| IBS file for GS864xxxxx
| Package: standard 209pin BGA
| DQ driver is programmable
| VDD=3.3V, VDDQ can be either 2.5V or 3.3V
| Date:   23 August 2006
| Rev.:
[IBIS Ver]   3.2
[File name]   gs864xxxxx.ibs
[File Rev]   1.0
[Date]   08/23/06
[Component]   GS864018T
[Manufacturer]   GSI Technology
[Package]
|  variable   typ   min   max
R_pkg   0.2   0.1   0.5
L_pkg   3nH   1nH   5nH
C_pkg   1.5pF   1pF   3pF
[Pin]   signal_name model_name  R_pin   L_pin   C_pin
 1   NC   NC
 2   NC   NC
 3   NC   NC
 4   VDDQ   POWER
 5   VSS   GND
 6   NC   NC
 7   NC   NC
 8   DQB1   IOBUF
 9   DQB2   IOBUF
 10   VSS   GND
 11   VDDQ   POWER
 12   DQB3   IOBUF
 13   DQB4   IOBUF
 14   FT#   INBUF
 15   VDD   POWER
 16   NC   NC
 17   VSS   GND
 18   DQB5   IOBUF
 19   DQB6   IOBUF
 20   VDDQ   POWER
 21   VSS   GND
 22   DQB7   IOBUF
 23   DQB8   IOBUF
 24   DQB9   IOBUF
 25   NC   NC
 26   VSS   GND
 27   VDDQ   POWER
 28   NC   NC
 29   NC   NC
 30   NC   NC
 31   LBO#   INBUF
 32   A5   INBUF
 33   A4   INBUF
 34   A3   INBUF
 35   A2   INBUF
 36   A1   INBUF
 37   A0   INBUF
 38   A20   INBUF
 39   A19   INBUF
 40   VSS   GND
 41   VDD   POWER
 42   A18   INBUF
 43   A17   INBUF
 44   A10   INBUF
 45   A11   INBUF
 46   A12   INBUF
 47   A13   INBUF
 48   A14   INBUF
 49   A15   INBUF
 50   A16   INBUF
 51   NC   NC
 52   NC   NC
 53   NC   NC
 54   VDDQ   POWER
 55   VSS   GND
 56   NC   NC
 57   NC   NC
 58   DQA1   IOBUF
 59   DQA2   IOBUF
 60   VSS   GND
 61   VDDQ   POWER
 62   DQA3   IOBUF
 63   DQA4   IOBUF
 64   ZZ   INBUF
 65   VDD   POWER
 66   NC   NC
 67   VSS   GND
 68   DQA5   IOBUF
 69   DQA6   IOBUF
 70   VDDQ   POWER
 71   VSS   GND
 72   DQA7   IOBUF
 73   DQA8   IOBUF
 74   DQA9   IOBUF
 75   NC   NC
 76   VSS   GND
 77   VDDQ   POWER
 78   NC   NC
 79   NC   NC
 80   A21   INBUF
 81   A9   INBUF
 82   A8   INBUF
 83   ADV#   INBUF
 84   ADSP#   INBUF
 85   ADSC#   INBUF
 86   G#   INBUF
 87   BW#   INBUF
 88   GW#   INBUF
 89   CK   INBUF
 90   VSS   GND
 91   VDD   POWER
 92   E3#   INBUF
 93   BA#   INBUF
 94   BB#   INBUF
 95   NC   NC
 96   NC   NC
 97   E2   INBUF
 98   E1#   INBUF
 99   A7   INBUF
 100   A6   INBUF
[Component]   GS864032T
[Manufacturer]   GSI Technology
[Package]
|  variable   typ   min   max
R_pkg   0.2   0.1   0.5
L_pkg   3nH   1nH   5nH
C_pkg   1.5pF   1pF   3pF
[Pin]   signal_name model_name  R_pin   L_pin   C_pin
 1   NC   NC
 2   DQC8   IOBUF
 3   DQC7   IOBUF
 4   VDDQ   POWER
 5   VSS   GND
 6   DQC6   IOBUF
 7   DQC5   IOBUF
 8   DQC4   IOBUF
 9   DQC3   IOBUF
 10   VSS   GND
 11   VDDQ   POWER
 12   DQC2   IOBUF
 13   DQC1   IOBUF
 14   FT#   INBUF
 15   VDD   POWER
 16   NC   NC
 17   VSS   GND
 18   DQD1   IOBUF
 19   DQD2   IOBUF
 20   VDDQ   POWER
 21   VSS   GND
 22   DQD3   IOBUF
 23   DQD4   IOBUF
 24   DQD5   IOBUF
 25   DQD6   IOBUF
 26   VSS   GND
 27   VDDQ   POWER
 28   DQD7   IOBUF
 29   DQD8   IOBUF
 30   NC   NC
 31   LBO#   INBUF
 32   A5   INBUF
 33   A4   INBUF
 34   A3   INBUF
 35   A2   INBUF
 36   A1   INBUF
 37   A0   INBUF
 38   A20   INBUF
 39   A19   INBUF
 40   VSS   GND
 41   VDD   POWER
 42   A18   INBUF
 43   A17   INBUF
 44   A10   INBUF
 45   A11   INBUF
 46   A12   INBUF
 47   A13   INBUF
 48   A14   INBUF
 49   A15   INBUF
 50   A16   INBUF
 51   NC   NC
 52   DQA8   IOBUF
 53   DQA7   IOBUF
 54   VDDQ   POWER
 55   VSS   GND
 56   DQA6   IOBUF
 57   DQA5   IOBUF
 58   DQA4   IOBUF
 59   DQA3   IOBUF
 60   VSS   GND
 61   VDDQ   POWER
 62   DQA2   IOBUF
 63   DQA1   IOBUF
 64   ZZ   INBUF
 65   VDD   POWER
 66   NC   NC
 67   VSS   GND
 68   DQB1   IOBUF
 69   DQB2   IOBUF
 70   VDDQ   POWER
 71   VSS   GND
 72   DQB3   IOBUF
 73   DQB4   IOBUF
 74   DQB5   IOBUF
 75   DQB6   IOBUF
 76   VSS   GND
 77   VDDQ   POWER
 78   DQB7   IOBUF
 79   DQB8   IOBUF
 80   NC   NC
 81   A9   INBUF
 82   A8   INBUF
 83   ADV#   INBUF
 84   ADSP#   INBUF
 85   ADSC#   INBUF
 86   G#   INBUF
 87   BW#   INBUF
 88   GW#   INBUF
 89   CK   INBUF
 90   VSS   GND
 91   VDD   POWER
 92   E3#   INBUF
 93   BA#   INBUF
 94   BB#   INBUF
 95   BC#   INBUF
 96   BD#   INBUF
 97   E2   INBUF
 98   E1#   INBUF
 99   A7   INBUF
 100   A6   INBUF
[Component]   GS864036t
[Manufacturer]   GSI Technology
[Package]
|  variable   typ   min   max
R_pkg   0.2   0.1   0.5
L_pkg   3nH   1nH   5nH
C_pkg   1.5pF   1pF   3pF
[Pin]   signal_name model_name  R_pin   L_pin   C_pin
 1   DQC9   IOBUF
 2   DQC8   IOBUF
 3   DQC7   IOBUF
 4   VDDQ   POWER
 5   VSS   GND
 6   DQC6   IOBUF
 7   DQC5   IOBUF
 8   DQC4   IOBUF
 9   DQC3   IOBUF
 10   VSS   GND
 11   VDDQ   POWER
 12   DQC2   IOBUF
 13   DQC1   IOBUF
 14   FT#   INBUF
 15   VDD   POWER
 16   NC   NC
 17   VSS   GND
 18   DQD1   IOBUF
 19   DQD2   IOBUF
 20   VDDQ   POWER
 21   VSS   GND
 22   DQD3   IOBUF
 23   DQD4   IOBUF
 24   DQD5   IOBUF
 25   DQD6   IOBUF
 26   VSS   GND
 27   VDDQ   POWER
 28   DQD7   IOBUF
 29   DQD8   IOBUF
 30   DQD9   IOBUF
 31   LBO#   INBUF
 32   A5   INBUF
 33   A4   INBUF
 34   A3   INBUF
 35   A2   INBUF
 36   A1   INBUF
 37   A0   INBUF
 38   A20   INBUF
 39   A19   INBUF
 40   VSS   GND
 41   VDD   POWER
 42   A18   INBUF
 43   A17   INBUF
 44   A10   INBUF
 45   A11   INBUF
 46   A12   INBUF
 47   A13   INBUF
 48   A14   INBUF
 49   A15   INBUF
 50   A16   INBUF
 51   DQA9   IOBUF
 52   DQA8   IOBUF
 53   DQA7   IOBUF
 54   VDDQ   POWER
 55   VSS   GND
 56   DQA6   IOBUF
 57   DQA5   IOBUF
 58   DQA4   IOBUF
 59   DQA3   IOBUF
 60   VSS   GND
 61   VDDQ   POWER
 62   DQA2   IOBUF
 63   DQA1   IOBUF
 64   ZZ   INBUF
 65   VDD   POWER
 66   NC   NC
 67   VSS   GND
 68   DQB1   IOBUF
 69   DQB2   IOBUF
 70   VDDQ   POWER
 71   VSS   GND
 72   DQB3   IOBUF
 73   DQB4   IOBUF
 74   DQB5   IOBUF
 75   DQB6   IOBUF
 76   VSS   GND
 77   VDDQ   POWER
 78   DQB7   IOBUF
 79   DQB8   IOBUF
 80   DQB9   IOBUF
 81   A9   INBUF
 82   A8   INBUF
 83   ADV#   INBUF
 84   ADSP#   INBUF
 85   ADSC#   INBUF
 86   G#   INBUF
 87   BW#   INBUF
 88   GW#   INBUF
 89   CK   INBUF
 90   VSS   GND
 91   VDD   POWER
 92   E3#   INBUF
 93   BA#   INBUF
 94   BB#   INBUF
 95   BC#   INBUF
 96   BD#   INBUF
 97   E2   INBUF
 98   E1#   INBUF
 99   A7   INBUF
 100   A6   INBUF
[Component]   GS8640E18T
[Manufacturer]   GSI Technology
[Package]
|  variable   typ   min   max
R_pkg   0.2   0.1   0.5
L_pkg   3nH   1nH   5nH
C_pkg   1.5pF   1pF   3pF
[Pin]   signal_name model_name  R_pin   L_pin   C_pin
 1   NC   NC
 2   NC   NC
 3   NC   NC
 4   VDDQ   POWER
 5   VSS   GND
 6   NC   NC
 7   NC   NC
 8   DQB1   IOBUF
 9   DQB2   IOBUF
 10   VSS   GND
 11   VDDQ   POWER
 12   DQB3   IOBUF
 13   DQB4   IOBUF
 14   FT#   INBUF
 15   VDD   POWER
 16   NC   NC
 17   VSS   GND
 18   DQB5   IOBUF
 19   DQB6   IOBUF
 20   VDDQ   POWER
 21   VSS   GND
 22   DQB7   IOBUF
 23   DQB8   IOBUF
 24   DQB9   IOBUF
 25   NC   NC
 26   VSS   GND
 27   VDDQ   POWER
 28   NC   NC
 29   NC   NC
 30   NC   NC
 31   LBO#   INBUF
 32   A5   INBUF
 33   A4   INBUF
 34   A3   INBUF
 35   A2   INBUF
 36   A1   INBUF
 37   A0   INBUF
 38   A20   INBUF
 39   A19   INBUF
 40   VSS   GND
 41   VDD   POWER
 42   A18   INBUF
 43   A17   INBUF
 44   A10   INBUF
 45   A11   INBUF
 46   A12   INBUF
 47   A13   INBUF
 48   A14   INBUF
 49   A15   INBUF
 50   A16   INBUF
 51   NC   NC
 52   NC   NC
 53   NC   NC
 54   VDDQ   POWER
 55   VSS   GND
 56   NC   NC
 57   NC   NC
 58   DQA1   IOBUF
 59   DQA2   IOBUF
 60   VSS   GND
 61   VDDQ   POWER
 62   DQA3   IOBUF
 63   DQA4   IOBUF
 64   ZZ   INBUF
 65   VDD   POWER
 66   NC   NC
 67   VSS   GND
 68   DQA5   IOBUF
 69   DQA6   IOBUF
 70   VDDQ   POWER
 71   VSS   GND
 72   DQA7   IOBUF
 73   DQA8   IOBUF
 74   DQA9   IOBUF
 75   NC   NC
 76   VSS   GND
 77   VDDQ   POWER
 78   NC   NC
 79   NC   NC
 80   A21   INBUF
 81   A9   INBUF
 82   A8   INBUF
 83   ADV#   INBUF
 84   ADSP#   INBUF
 85   ADSC#   INBUF
 86   G#   INBUF
 87   BW#   INBUF
 88   GW#   INBUF
 89   CK   INBUF
 90   VSS   GND
 91   VDD   POWER
 92   E3#   INBUF
 93   BA#   INBUF
 94   BB#   INBUF
 95   NC   NC
 96   NC   NC
 97   E2   INBUF
 98   E1#   INBUF
 99   A7   INBUF
 100   A6   INBUF
[Component]   GS8640E32T
[Manufacturer]   GSI Technology
[Package]
|  variable   typ   min   max
R_pkg   0.2   0.1   0.5
L_pkg   3nH   1nH   5nH
C_pkg   1.5pF   1pF   3pF
[Pin]   signal_name model_name  R_pin   L_pin   C_pin
 1   NC   NC
 2   DQC8   IOBUF
 3   DQC7   IOBUF
 4   VDDQ   POWER
 5   VSS   GND
 6   DQC6   IOBUF
 7   DQC5   IOBUF
 8   DQC4   IOBUF
 9   DQC3   IOBUF
 10   VSS   GND
 11   VDDQ   POWER
 12   DQC2   IOBUF
 13   DQC1   IOBUF
 14   FT#   INBUF
 15   VDD   POWER
 16   NC   NC
 17   VSS   GND
 18   DQD1   IOBUF
 19   DQD2   IOBUF
 20   VDDQ   POWER
 21   VSS   GND
 22   DQD3   IOBUF
 23   DQD4   IOBUF
 24   DQD5   IOBUF
 25   DQD6   IOBUF
 26   VSS   GND
 27   VDDQ   POWER
 28   DQD7   IOBUF
 29   DQD8   IOBUF
 30   NC   NC
 31   LBO#   INBUF
 32   A5   INBUF
 33   A4   INBUF
 34   A3   INBUF
 35   A2   INBUF
 36   A1   INBUF
 37   A0   INBUF
 38   A20   INBUF
 39   A19   INBUF
 40   VSS   GND
 41   VDD   POWER
 42   A18   INBUF
 43   A17   INBUF
 44   A10   INBUF
 45   A11   INBUF
 46   A12   INBUF
 47   A13   INBUF
 48   A14   INBUF
 49   A15   INBUF
 50   A16   INBUF
 51   NC   NC
 52   DQA8   IOBUF
 53   DQA7   IOBUF
 54   VDDQ   POWER
 55   VSS   GND
 56   DQA6   IOBUF
 57   DQA5   IOBUF
 58   DQA4   IOBUF
 59   DQA3   IOBUF
 60   VSS   GND
 61   VDDQ   POWER
 62   DQA2   IOBUF
 63   DQA1   IOBUF
 64   ZZ   INBUF
 65   VDD   POWER
 66   NC   NC
 67   VSS   GND
 68   DQB1   IOBUF
 69   DQB2   IOBUF
 70   VDDQ   POWER
 71   VSS   GND
 72   DQB3   IOBUF
 73   DQB4   IOBUF
 74   DQB5   IOBUF
 75   DQB6   IOBUF
 76   VSS   GND
 77   VDDQ   POWER
 78   DQB7   IOBUF
 79   DQB8   IOBUF
 80   NC   NC
 81   A9   INBUF
 82   A8   INBUF
 83   ADV#   INBUF
 84   ADSP#   INBUF
 85   ADSC#   INBUF
 86   G#   INBUF
 87   BW#   INBUF
 88   GW#   INBUF
 89   CK   INBUF
 90   VSS   GND
 91   VDD   POWER
 92   E3#   INBUF
 93   BA#   INBUF
 94   BB#   INBUF
 95   BC#   INBUF
 96   BD#   INBUF
 97   E2   INBUF
 98   E1#   INBUF
 99   A7   INBUF
 100   A6   INBUF
[Component]   GS8640E36t
[Manufacturer]   GSI Technology
[Package]
|  variable   typ   min   max
R_pkg   0.2   0.1   0.5
L_pkg   3nH   1nH   5nH
C_pkg   1.5pF   1pF   3pF
[Pin]   signal_name model_name  R_pin   L_pin   C_pin
 1   DQC9   IOBUF
 2   DQC8   IOBUF
 3   DQC7   IOBUF
 4   VDDQ   POWER
 5   VSS   GND
 6   DQC6   IOBUF
 7   DQC5   IOBUF
 8   DQC4   IOBUF
 9   DQC3   IOBUF
 10   VSS   GND
 11   VDDQ   POWER
 12   DQC2   IOBUF
 13   DQC1   IOBUF
 14   FT#   INBUF
 15   VDD   POWER
 16   NC   NC
 17   VSS   GND
 18   DQD1   IOBUF
 19   DQD2   IOBUF
 20   VDDQ   POWER
 21   VSS   GND
 22   DQD3   IOBUF
 23   DQD4   IOBUF
 24   DQD5   IOBUF
 25   DQD6   IOBUF
 26   VSS   GND
 27   VDDQ   POWER
 28   DQD7   IOBUF
 29   DQD8   IOBUF
 30   DQD9   IOBUF
 31   LBO#   INBUF
 32   A5   INBUF
 33   A4   INBUF
 34   A3   INBUF
 35   A2   INBUF
 36   A1   INBUF
 37   A0   INBUF
 38   A20   INBUF
 39   A19   INBUF
 40   VSS   GND
 41   VDD   POWER
 42   A18   INBUF
 43   A17   INBUF
 44   A10   INBUF
 45   A11   INBUF
 46   A12   INBUF
 47   A13   INBUF
 48   A14   INBUF
 49   A15   INBUF
 50   A16   INBUF
 51   DQA9   IOBUF
 52   DQA8   IOBUF
 53   DQA7   IOBUF
 54   VDDQ   POWER
 55   VSS   GND
 56   DQA6   IOBUF
 57   DQA5   IOBUF
 58   DQA4   IOBUF
 59   DQA3   IOBUF
 60   VSS   GND
 61   VDDQ   POWER
 62   DQA2   IOBUF
 63   DQA1   IOBUF
 64   ZZ   INBUF
 65   VDD   POWER
 66   NC   NC
 67   VSS   GND
 68   DQB1   IOBUF
 69   DQB2   IOBUF
 70   VDDQ   POWER
 71   VSS   GND
 72   DQB3   IOBUF
 73   DQB4   IOBUF
 74   DQB5   IOBUF
 75   DQB6   IOBUF
 76   VSS   GND
 77   VDDQ   POWER
 78   DQB7   IOBUF
 79   DQB8   IOBUF
 80   DQB9   IOBUF
 81   A9   INBUF
 82   A8   INBUF
 83   ADV#   INBUF
 84   ADSP#   INBUF
 85   ADSC#   INBUF
 86   G#   INBUF
 87   BW#   INBUF
 88   GW#   INBUF
 89   CK   INBUF
 90   VSS   GND
 91   VDD   POWER
 92   E3#   INBUF
 93   BA#   INBUF
 94   BB#   INBUF
 95   BC#   INBUF
 96   BD#   INBUF
 97   E2   INBUF
 98   E1#   INBUF
 99   A7   INBUF
 100   A6   INBUF
[Component]   GS864218B
[Manufacturer]   GSI Technology
[Package]
|  variable   typ   min   max
R_pkg   0.2   0.1   0.5
L_pkg   3nH   1nH   5nH
C_pkg   1.5pF   1pF   3pF
[Pin]   signal_name model_name  R_pin   L_pin   C_pin
 A1   VDDQ   POWER
 A2   A6   INBUF
 A3   A7   INBUF
 A4   ADSP#   INBUF
 A5   A8   INBUF
 A6   A9   INBUF
 A7   VDDQ   POWER
 B1   NC   NC
 B2   A18   INBUF
 B3   A4   INBUF
 B4   ADSC#   INBUF
 B5   A15   INBUF
 B6   A17   INBUF
 B7   NC   NC
 C1   NC   NC
 C2   A5   INBUF
 C3   A3   INBUF
 C4   VDD   POWER
 C5   A14   INBUF
 C6   A16   INBUF
 C7   NC   NC
 D1   DQB1   Progbuf1
 D2   NC   NC
 D3   VSS   GND
 D4   ZQ   INBUF
 D5   VSS   GND
 D6   DQA9   Progbuf1
 D7   NC   NC
 E1   NC   NC
 E2   DQB2   Progbuf1
 E3   VSS   GND
 E4   E1#   INBUF
 E5   VSS   GND
 E6   NC   NC
 E7   DQA8   Progbuf1
 F1   VDDQ   POWER
 F2   NC   NC
 F3   VSS   GND
 F4   G#   INBUF
 F5   VSS   GND
 F6   DQA7   Progbuf1
 F7   VDDQ   POWER
 G1   NC   NC
 G2   DQB3   Progbuf1
 G3   BB#   INBUF
 G4   ADV#   INBUF
 G5   NC   NC
 G6   NC   NC
 G7   DQA6   Progbuf1
 H1   DQB4   Progbuf1
 H2   NC   NC
 H3   VSS   GND
 H4   GW#   INBUF
 H5   VSS   GND
 H6   DQA5   Progbuf1
 H7   NC   NC
 J1   VDDQ   POWER
 J2   VDD   POWER
 J3   NC   NC
 J4   VDD   POWER
 J5   NC   NC
 J6   VDD   POWER
 J7   VDDQ   POWER
 K1   NC   NC
 K2   DQB5   Progbuf1
 K3   VSS   GND
 K4   CK   INBUF
 K5   VSS   GND
 K6   NC   NC
 K7   DQA4   Progbuf1
 L1   DQB6   Progbuf1
 L2   NC   NC
 L3   NC   NC
 L4   SCD   INBUF
 L5   BA#   INBUF
 L6   DQA3   Progbuf1
 L7   NC   NC
 M1   VDDQ   POWER
 M2   DQB7   Progbuf1
 M3   VSS   GND
 M4   BW#   INBUF
 M5   VSS   GND
 M6   NC   NC
 M7   VDDQ   POWER
 N1   DQB8   Progbuf1
 N2   NC   NC
 N3   VSS   GND
 N4   A1   INBUF
 N5   VSS   GND
 N6   DQA2   Progbuf1
 N7   NC   NC
 P1   NC   NC
 P2   DQB9   Progbuf1
 P3   VSS   GND
 P4   A0   INBUF
 P5   VSS   GND
 P6   NC   NC
 P7   DQA1   Progbuf1
 R1   NC   NC
 R2   A2   INBUF
 R3   LBO#   INBUF
 R4   VDD   POWER
 R5   FT#   INBUF
 R6   A13   INBUF
 R7   NC   NC
 T1   A20   INBUF
 T2   A10   INBUF
 T3   A11   INBUF
 T4   A21   INBUF
 T5   A12   INBUF
 T6   A19   INBUF
 T7   ZZ   INBUF
 U1   VDDQ   POWER
 U2   TMS   INBUF
 U3   TDI   INBUF
 U4   TCK   INBUF
 U5   TDO   Progbuf2
 U6   NC   NC
 U7   VDDQ   POWER
[Component]   GS864236B
[Manufacturer]   GSI Technology
[Package]
|  variable   typ   min   max
R_pkg   0.2   0.1   0.5
L_pkg   3nH   1nH   5nH
C_pkg   1.5pF   1pF   3pF
[Pin]   signal_name model_name  R_pin   L_pin   C_pin
 A1   VDDQ   POWER
 A2   A6   INBUF
 A3   A7   INBUF
 A4   ADSP#   INBUF
 A5   A8   INBUF
 A6   A9   INBUF
 A7   VDDQ   POWER
 B1   NC   NC
 B2   A18   INBUF
 B3   A4   INBUF
 B4   ADSC#   INBUF
 B5   A15   INBUF
 B6   A17   INBUF
 B7   NC   NC
 C1   NC   NC
 C2   A5   INBUF
 C3   A3   INBUF
 C4   VDD   POWER
 C5   A14   INBUF
 C6   A16   INBUF
 C7   NC   NC
 D1   DQc4   Progbuf1
 D2   DQC9   Progbuf1
 D3   VSS   GND
 D4   ZQ   INBUF
 D5   VSS   GND
 D6   DQB9   Progbuf1
 D7   DQB4   Progbuf1
 E1   DQc3   Progbuf1
 E2   DQC8   Progbuf1
 E3   VSS   GND
 E4   E1#   INBUF
 E5   VSS   GND
 E6   DQB8   Progbuf1
 E7   DQB3   Progbuf1
 F1   VDDQ   POWER
 F2   DQC7   Progbuf1
 F3   VSS   GND
 F4   G#   INBUF
 F5   VSS   GND
 F6   DQB7   Progbuf1
 F7   VDDQ   POWER
 G1   DQc2   Progbuf1
 G2   DQC6   Progbuf1
 G3   BC#   INBUF
 G4   ADV#   INBUF
 G5   BB#   INBUF
 G6   DQB6   Progbuf1
 G7   DQB2   Progbuf1
 H1   DQc1   Progbuf1
 H2   DQC5   Progbuf1
 H3   VSS   GND
 H4   GW#   INBUF
 H5   VSS   GND
 H6   DQB5   Progbuf1
 H7   DQB1   Progbuf1
 J1   VDDQ   POWER
 J2   VDD   POWER
 J3   NC   NC
 J4   VDD   POWER
 J5   NC   NC
 J6   VDD   POWER
 J7   VDDQ   POWER
 K1   DQD1   Progbuf1
 K2   DQD5   Progbuf1
 K3   VSS   GND
 K4   CK   INBUF
 K5   VSS   GND
 K6   DQA5   Progbuf1
 K7   DQA1   Progbuf1
 L1   DQD2   Progbuf1
 L2   DQD6   Progbuf1
 L3   BD#   INBUF
 L4   SCD   INBUF
 L5   BA#   INBUF
 L6   DQA6   Progbuf1
 L7   DQA2   Progbuf1
 M1   VDDQ   POWER
 M2   DQD7   Progbuf1
 M3   VSS   GND
 M4   BW#   INBUF
 M5   VSS   GND
 M6   DQA7   Progbuf1
 M7   VDDQ   POWER
 N1   DQD3   Progbuf1
 N2   DQD8   Progbuf1
 N3   VSS   GND
 N4   A1   INBUF
 N5   VSS   GND
 N6   DQA8   Progbuf1
 N7   DQA3   Progbuf1
 P1   DQD4   Progbuf1
 P2   DQD9   Progbuf1
 P3   VSS   GND
 P4   A0   INBUF
 P5   VSS   GND
 P6   DQA9   Progbuf1
 P7   DQA4   Progbuf1
 R1   NC   NC
 R2   A2   INBUF
 R3   LBO#   INBUF
 R4   VDD   POWER
 R5   FT#   INBUF
 R6   A13   INBUF
 R7   NC   NC
 T1   NC   NC
 T2   A20   INBUF
 T3   A10   INBUF
 T4   A11   INBUF
 T5   A12   INBUF
 T6   A20   INBUF
 T7   ZZ   INBUF
 U1   VDDQ   POWER
 U2   TMS   INBUF
 U3   TDI   INBUF
 U4   TCK   INBUF
 U5   TDO   Progbuf2
 U6   NC   NC
 U7   VDDQ   POWER
[Component]   GS864272C
[Manufacturer]   GSI Technology
[Package]
|  variable   typ   min   max
R_pkg   0.2   0.1   0.5
L_pkg   3nH   1nH   5nH
C_pkg   1.5pF   1pF   3pF
[Pin]   signal_name model_name  R_pin   L_pin   C_pin
 A1   DQG5   Progbuf1
 A2   DQG1   Progbuf1
 A3   A15   INBUF
 A4   E2   INBUF
 A5   ADSP   INBUF
 A6   ADSC   INBUF
 A7   ADV   INBUF
 A8   E3   INBUF
 A9   A17   INBUF
 A10   DQB1   Progbuf1
 A11   DQB5   Progbuf1
 B1   DQG6   Progbuf1
 B2   DQG2   Progbuf1
 B3   BC   INBUF
 B4   BG   INBUF
 B5   NC   NC
 B6   BW   INBUF
 B7   A16   INBUF
 B8   BB   INBUF
 B9   BF   INBUF
 B10   DQB2   Progbuf1
 B11   DQB6   Progbuf1
 C1   DQG7   Progbuf1
 C2   DQG3   Progbuf1
 C3   BH   INBUF
 C4   BD   INBUF
 C5   NC   NC
 C6   E1   INBUF
 C7   NC   NC
 C8   BE   INBUF
 C9   BA   INBUF
 C10   DQB3   Progbuf1
 C11   DQB7   Progbuf1
 D1   DQG8   Progbuf1
 D2   DQG4   Progbuf1
 D3   VSS   GND
 D4   NC   NC
 D5   NC   NC
 D6   G   INBUF
 D7   GW   INBUF
 D8   NC   NC
 D9   VSS   GND
 D10   DQB4   Progbuf1
 D11   DQB8   Progbuf1
 E1   DQG9   Progbuf1
 E2   DQC9   Progbuf1
 E3   VDDQ   POWER
 E4   VDDQ   POWER
 E5   VDD   POWER
 E6   VDD   POWER
 E7   VDD   POWER
 E8   VDDQ   POWER
 E9   VDDQ   POWER
 E10   DQF9   Progbuf1
 E11   DQB9   Progbuf1
 F1   DQC4   Progbuf1
 F2   DQC8   Progbuf1
 F3   VSS   GND
 F4   VSS   GND
 F5   VSS   GND
 F6   ZQ   INBUF
 F7   VSS   GND
 F8   VSS   GND
 F9   VSS   GND
 F10   DQF8   Progbuf1
 F11   DQF4   Progbuf1
 G1   DQC3   Progbuf1
 G2   DQC7   Progbuf1
 G3   VDDQ   POWER
 G4   VDDQ   POWER
 G5   VDD   POWER
 G6   MCH   INBUF
 G7   VDD   POWER
 G8   VDDQ   POWER
 G9   VDDQ   POWER
 G10   DQF7   Progbuf1
 G11   DQF3   Progbuf1
 H1   DQC2   Progbuf1
 H2   DQC6   Progbuf1
 H3   VSS   GND
 H4   VSS   GND
 H5   VSS   GND
 H6   MCL   INBUF
 H7   VSS   GND
 H8   VSS   GND
 H9   VSS   GND
 H10   DQF6   Progbuf1
 H11   DQF2   Progbuf1
 J1   DQC1   Progbuf1
 J2   DQC5   Progbuf1
 J3   VDDQ   POWER
 J4   VDDQ   POWER
 J5   VDD   POWER
 J6   MCL   INBUF
 J7   VDD   POWER
 J8   VDDQ   POWER
 J9   VDDQ   POWER
 J10   DQF5   Progbuf1
 J11   DQF1   Progbuf1
 K1   NC   NC
 K2   NC   NC
 K3   CK   INBUF
 K4   NC   NC
 K5   VSS   GND
 K6   MCL   INBUF
 K7   VSS   GND
 K8   NC   NC
 K9   NC   NC
 K10   NC   NC
 K11   NC   NC
 L1   DQH1   Progbuf1
 L2   DQH5   Progbuf1
 L3   VDDQ   POWER
 L4   VDDQ   POWER
 L5   VDD   POWER
 L6   FT   INBUF
 L7   VDD   POWER
 L8   VDDQ   POWER
 L9   VDDQ   POWER
 L10   DQA5   Progbuf1
 L11   DQA1   Progbuf1
 M1   DQH2   Progbuf1
 M2   DQH6   Progbuf1
 M3   VSS   GND
 M4   VSS   GND
 M5   VSS   GND
 M6   MCL   INBUF
 M7   VSS   GND
 M8   VSS   GND
 M9   VSS   GND
 M10   DQA6   Progbuf1
 M11   DQA2   Progbuf1
 N1   DQH3   Progbuf1
 N2   DQH7   Progbuf1
 N3   VDDQ   POWER
 N4   VDDQ   POWER
 N5   VDD   POWER
 N6   SCD   INBUF
 N7   VDD   POWER
 N8   VDDQ   POWER
 N9   VDDQ   POWER
 N10   DQA7   Progbuf1
 N11   DQA3   Progbuf1
 P1   DQH4   Progbuf1
 P2   DQH8   Progbuf1
 P3   VSS   GND
 P4   VSS   GND
 P5   VSS   GND
 P6   ZZ   INBUF
 P7   VSS   GND
 P8   VSS   GND
 P9   VSS   GND
 P10   DQA8   Progbuf1
 P11   DQA4   Progbuf1
 R1   DQD9   Progbuf1
 R2   DQH9   Progbuf1
 R3   VDDQ   POWER
 R4   VDDQ   POWER
 R5   VDD   POWER
 R6   VDD   POWER
 R7   VDD   POWER
 R8   VDDQ   POWER
 R9   VDDQ   POWER
 R10   DQA9   Progbuf1
 R11   DQE9   Progbuf1
 T1   DQD8   Progbuf1
 T2   DQD4   Progbuf1
 T3   VSS   GND
 T4   NC   NC
 T5   NC   NC
 T6   LBO   INBUF
 T7   NC   NC
 T8   NC   NC
 T9   VSS   GND
 T10   DQE4   Progbuf1
 T11   DQE8   Progbuf1
 U1   DQD7   Progbuf1
 U2   DQD3   Progbuf1
 U3   A19   INBUF
 U4   A14   INBUF
 U5   A13   INBUF
 U6   A12   INBUF
 U7   A11   INBUF
 U8   A10   INBUF
 U9   A18   INBUF
 U10   DQE3   Progbuf1
 U11   DQE7   Progbuf1
 V1   DQD6   Progbuf1
 V2   DQD2   Progbuf1
 V3   A9   INBUF
 V4   A8   INBUF
 V5   A7   INBUF
 V6   A1   INBUF
 V7   A6   INBUF
 V8   A5   INBUF
 V9   A4   INBUF
 V10   DQE2   Progbuf1
 V11   DQE6   Progbuf1
 W1   DQD5   Progbuf1
 W2   DQD1   Progbuf1
 W3   TMS   INBUF
 W4   TDI   INBUF
 W5   A3   INBUF
 W6   A0   INBUF
 W7   A2   INBUF
 W8   TDO   Progbuf2
 W9   TCK   INBUF
 W10   DQE1   Progbuf1
 W11   DQE5   Progbuf1
[Component]   GS8640FZ18T
[Manufacturer]   GSI Technology
[Package]
|  variable   typ   min   max
R_pkg   0.2   0.1   0.5
L_pkg   3nH   1nH   5nH
C_pkg   1.5pF   1pF   3pF
[Pin]   signal_name model_name  R_pin   L_pin   C_pin
 1   NC   NC
 2   NC   NC
 3   NC   NC
 4   VDDQ   POWER
 5   VSS   GND
 6   NC   NC
 7   NC   NC
 8   DQB1   IOBUF
 9   DQB2   IOBUF
 10   VSS   GND
 11   VDDQ   POWER
 12   DQB3   IOBUF
 13   DQB4   IOBUF
 14   NC   NC
 15   VDD   POWER
 16   NC   NC
 17   VSS   GND
 18   DQB5   IOBUF
 19   DQB6   IOBUF
 20   VDDQ   POWER
 21   VSS   GND
 22   DQB7   IOBUF
 23   DQB8   IOBUF
 24   DQB9   IOBUF
 25   NC   NC
 26   VSS   GND
 27   VDDQ   POWER
 28   NC   NC
 29   NC   NC
 30   NC   NC
 31   LBO#   INBUF
 32   A5   INBUF
 33   A4   INBUF
 34   A3   INBUF
 35   A2   INBUF
 36   A1   INBUF
 37   A0   INBUF
 38   NC   NC
 39   NC   NC
 40   VSS   GND
 41   VDD   POWER
 42   A20   INBUF
 43   A19   INBUF
 44   A10   INBUF
 45   A11   INBUF
 46   A12   INBUF
 47   A13   INBUF
 48   A14   INBUF
 49   A15   INBUF
 50   A16   INBUF
 51   NC   NC
 52   NC   NC
 53   NC   NC
 54   VDDQ   POWER
 55   VSS   GND
 56   DQA6   IOBUF
 57   NC   NC
 58   DQA1   IOBUF
 59   DQA2   IOBUF
 60   VSS   GND
 61   VDDQ   POWER
 62   DQA3   IOBUF
 63   DQA4   IOBUF
 64   ZZ   INBUF
 65   VDD   POWER
 66   NC   NC
 67   VSS   GND
 68   DQA5   IOBUF
 69   DQA6   IOBUF
 70   VDDQ   POWER
 71   VSS   GND
 72   DQA7   IOBUF
 73   DQA8   IOBUF
 74   DQA9   IOBUF
 75   NC   NC
 76   VSS   GND
 77   VDDQ   POWER
 78   NC   NC
 79   NC   NC
 80   A21   INBUF
 81   A9   INBUF
 82   A8   INBUF
 83   A17   INBUF
 84   A18   INBUF
 85   ADV   INBUF
 86   G#   INBUF
 87   CKE#   INBUF
 88   W#   INBUF
 89   CK   INBUF
 90   VSS   GND
 91   VDD   POWER
 92   E3#   INBUF
 93   BA#   INBUF
 94   BB#   INBUF
 95   NC   NC
 96   NC   NC
 97   E2   INBUF
 98   E1#   INBUF
 99   A7   INBUF
 100   A6   INBUF
[Component]   GS8640FZ36T
[Manufacturer]   GSI Technology
[Package]
|  variable   typ   min   max
R_pkg   0.2   0.1   0.5
L_pkg   3nH   1nH   5nH
C_pkg   1.5pF   1pF   3pF
[Pin]   signal_name model_name  R_pin   L_pin   C_pin
  1   DQC9   IOBUF
  2   DQC8   IOBUF
  3   DQC7   IOBUF
  4   VDDQ   POWER
  5   VSS   GND
  6   DQC6   IOBUF
  7   DQC5   IOBUF
  8   DQC4   IOBUF
  9   DQC3   IOBUF
 10   VSS   GND
 11   VDDQ   POWER
 12   DQC2   IOBUF
 13   DQC1   IOBUF
 14   NC   NC
 15   VDD   POWER
 16   NC   NC
 17   VSS   GND
 18   DQD1   IOBUF
 19   DQD2   IOBUF
 20   VDDQ   POWER
 21   VSS   GND
 22   DQD3   IOBUF
 23   DQD4   IOBUF
 24   DQD5   IOBUF
 25   DQD6   IOBUF
 26   VSS   GND
 27   VDDQ   POWER
 28   DQD7   IOBUF
 29   DQD8   IOBUF
 30   DQD9   IOBUF
 31   NLBO   INBUF
 32   A5   INBUF
 33   A4   INBUF
 34   A3   INBUF
 35   A2   INBUF
 36   A1   INBUF
 37   A0   INBUF
 38   NC   NC
 39   NC   NC
 40   VSS   POWER
 41   VDD   POWER
 42   A6   INBUF
 43   A7   INBUF
 44   A8   INBUF
 45   A9   INBUF
 46   A10   INBUF
 47   A11   INBUF
 48   A12   INBUF
 49   A13   INBUF
 50   A14   INBUF
 51   DQA1   IOBUF
 52   DQA2   IOBUF
 53   DQA3   IOBUF
 54   VDDQ   POWER
 55   VSS   GND
 56   DQA4   IOBUF
 57   DQA5   IOBUF
 58   DQA6   IOBUF
 59   DQA7   IOBUF
 60   VSS   GND
 61   VDDQ   POWER
 62   DQA8   IOBUF
 63   DQA9   IOBUF
 64   ZZ   INBUF
 65   VDD   POWER
 66   NC   NC
 67   VSS   GND
 68   DQB1   IOBUF
 69   DQB2   IOBUF
 70   VDDQ   POWER
 71   VSS   GND
 72   DQB3   IOBUF
 73   DQB4   IOBUF
 74   DQB5   IOBUF
 75   DQB6   IOBUF
 76   VSS   GND
 77   VDDQ   POWER
 78   DQB7   IOBUF
 79   DQB8   IOBUF
 80   DQB9   IOBUF
 81   A15   INBUF
 82   A16   INBUF
 83   A17   INBUF
 84   A18   INBUF
 85   ADV   INBUF
 86   NG   INBUF
 87   NCKE   INBUF
 88   NW   INBUF
 89   CK   INBUF
 90   VSS   GND
 91   VDD   POWER
 92   NE3   INBUF
 93   NBA   INBUF
 94   NBB   INBUF
 95   NBC   INBUF
 96   NBD   INBUF
 97   E2   INBUF
 98   NE1   INBUF
 99   A19   INBUF
100   A20   INBUF
[Component]   GS8640Z18T
[Manufacturer]   GSI Technology
[Package]
|  variable   typ   min   max
R_pkg   0.2   0.1   0.5
L_pkg   3nH   1nH   5nH
C_pkg   1.5pF   1pF   3pF
[Pin]   signal_name model_name  R_pin   L_pin   C_pin
 1   NC   NC
 2   NC   NC
 3   NC   NC
 4   VDDQ   POWER
 5   VSS   GND
 6   NC   NC
 7   NC   NC
 8   DQB1   IOBUF
 9   DQB2   IOBUF
 10   VSS   GND
 11   VDDQ   POWER
 12   DQB3   IOBUF
 13   DQB4   IOBUF
 14   FT#   INBUF
 15   VDD   POWER
 16   NC   NC
 17   VSS   GND
 18   DQB5   IOBUF
 19   DQB6   IOBUF
 20   VDDQ   POWER
 21   VSS   GND
 22   DQB7   IOBUF
 23   DQB8   IOBUF
 24   DQB9   IOBUF
 25   NC   NC
 26   VSS   GND
 27   VDDQ   POWER
 28   NC   NC
 29   NC   NC
 30   NC   NC
 31   LBO#   INBUF
 32   A5   INBUF
 33   A4   INBUF
 34   A3   INBUF
 35   A2   INBUF
 36   A1   INBUF
 37   A0   INBUF
 38   NC   NC
 39   NC   NC
 40   VSS   GND
 41   VDD   POWER
 42   A20   INBUF
 43   A19   INBUF
 44   A10   INBUF
 45   A11   INBUF
 46   A12   INBUF
 47   A13   INBUF
 48   A14   INBUF
 49   A15   INBUF
 50   A16   INBUF
 51   NC   NC
 52   NC   NC
 53   NC   NC
 54   VDDQ   POWER
 55   VSS   GND
 56   DQA6   IOBUF
 57   NC   NC
 58   DQA1   IOBUF
 59   DQA2   IOBUF
 60   VSS   GND
 61   VDDQ   POWER
 62   DQA3   IOBUF
 63   DQA4   IOBUF
 64   ZZ   INBUF
 65   VDD   POWER
 66   NC   NC
 67   VSS   GND
 68   DQA5   IOBUF
 69   DQA6   IOBUF
 70   VDDQ   POWER
 71   VSS   GND
 72   DQA7   IOBUF
 73   DQA8   IOBUF
 74   DQA9   IOBUF
 75   NC   NC
 76   VSS   GND
 77   VDDQ   POWER
 78   NC   NC
 79   NC   NC
 80   A21   INBUF
 81   A9   INBUF
 82   A8   INBUF
 83   A17   INBUF
 84   A18   INBUF
 85   ADV   INBUF
 86   G#   INBUF
 87   CKE#   INBUF
 88   W#   INBUF
 89   CK   INBUF
 90   VSS   GND
 91   VDD   POWER
 92   E3#   INBUF
 93   BA#   INBUF
 94   BB#   INBUF
 95   NC   NC
 96   NC   NC
 97   E2   INBUF
 98   E1#   INBUF
 99   A7   INBUF
 100   A6   INBUF
[Component]   GS8640Z36T
[Manufacturer]   GSI Technology
[Package]
|  variable   typ   min   max
R_pkg   0.2   0.1   0.5
L_pkg   3nH   1nH   5nH
C_pkg   1.5pF   1pF   3pF
[Pin]   signal_name model_name  R_pin   L_pin   C_pin
  1   DQC9   IOBUF
  2   DQC8   IOBUF
  3   DQC7   IOBUF
  4   VDDQ   POWER
  5   VSS   GND
  6   DQC6   IOBUF
  7   DQC5   IOBUF
  8   DQC4   IOBUF
  9   DQC3   IOBUF
 10   VSS   GND
 11   VDDQ   POWER
 12   DQC2   IOBUF
 13   DQC1   IOBUF
 14   NFT   INBUF
 15   VDD   POWER
 16   NC   NC
 17   VSS   GND
 18   DQD1   IOBUF
 19   DQD2   IOBUF
 20   VDDQ   POWER
 21   VSS   GND
 22   DQD3   IOBUF
 23   DQD4   IOBUF
 24   DQD5   IOBUF
 25   DQD6   IOBUF
 26   VSS   GND
 27   VDDQ   POWER
 28   DQD7   IOBUF
 29   DQD8   IOBUF
 30   DQD9   IOBUF
 31   NLBO   INBUF
 32   A5   INBUF
 33   A4   INBUF
 34   A3   INBUF
 35   A2   INBUF
 36   A1   INBUF
 37   A0   INBUF
 38   NC   NC
 39   NC   NC
 40   VSS   POWER
 41   VDD   POWER
 42   A6   INBUF
 43   A7   INBUF
 44   A8   INBUF
 45   A9   INBUF
 46   A10   INBUF
 47   A11   INBUF
 48   A12   INBUF
 49   A13   INBUF
 50   A14   INBUF
 51   DQA1   IOBUF
 52   DQA2   IOBUF
 53   DQA3   IOBUF
 54   VDDQ   POWER
 55   VSS   GND
 56   DQA4   IOBUF
 57   DQA5   IOBUF
 58   DQA6   IOBUF
 59   DQA7   IOBUF
 60   VSS   GND
 61   VDDQ   POWER
 62   DQA8   IOBUF
 63   DQA9   IOBUF
 64   ZZ   INBUF
 65   VDD   POWER
 66   NC   NC
 67   VSS   GND
 68   DQB1   IOBUF
 69   DQB2   IOBUF
 70   VDDQ   POWER
 71   VSS   GND
 72   DQB3   IOBUF
 73   DQB4   IOBUF
 74   DQB5   IOBUF
 75   DQB6   IOBUF
 76   VSS   GND
 77   VDDQ   POWER
 78   DQB7   IOBUF
 79   DQB8   IOBUF
 80   DQB9   IOBUF
 81   A15   INBUF
 82   A16   INBUF
 83   A17   INBUF
 84   A18   INBUF
 85   ADV   INBUF
 86   NG   INBUF
 87   NCKE   INBUF
 88   NW   INBUF
 89   CK   INBUF
 90   VSS   GND
 91   VDD   POWER
 92   NE3   INBUF
 93   NBA   INBUF
 94   NBB   INBUF
 95   NBC   INBUF
 96   NBD   INBUF
 97   E2   INBUF
 98   NE1   INBUF
 99   A19   INBUF
100   A20   INBUF
[Component]   GS8642Z18B
[Manufacturer]   GSI Technology
[Package]
|  variable   typ   min   max
R_pkg   0.2   0.1   0.5
L_pkg   3nH   1nH   5nH
C_pkg   1.5pF   1pF   3pF
[Pin]   signal_name model_name  R_pin   L_pin   C_pin
 A1   VDDQ   POWER
 A2   A6   INBUF
 A3   A7   INBUF
 A4   A18   INBUF
 A5   A8   INBUF
 A6   A9   INBUF
 A7   VDDQ   POWER
 B1   NC   NC
 B2   E2   INBUF
 B3   A4   INBUF
 B4   ADV   INBUF
 B5   A15   INBUF
 B6   E3#   INBUF
 B7   NC   NC
 C1   NC   NC
 C2   A5   INBUF
 C3   A3   INBUF
 C4   VDD   POWER
 C5   A14   INBUF
 C6   A16   INBUF
 C7   NC   NC
 D1   DQB1   Progbuf1
 D2   NC   NC
 D3   VSS   GND
 D4   ZQ   INBUF
 D5   VSS   GND
 D6   DQA9   Progbuf1
 D7   NC   NC
 E1   NC   NC
 E2   DQB2   Progbuf1
 E3   VSS   GND
 E4   E1#   INBUF
 E5   VSS   GND
 E6   NC   NC
 E7   DQA8   Progbuf1
 F1   VDDQ   POWER
 F2   NC   NC
 F3   VSS   GND
 F4   G#   INBUF
 F5   VSS   GND
 F6   DQA7   Progbuf1
 F7   VDDQ   POWER
 G1   NC   NC
 G2   DQB3   Progbuf1
 G3   BB#   INBUF
 G4   A17   INBUF
 G5   NC   NC
 G6   NC   NC
 G7   NC   NC
 H1   DQB4   Progbuf1
 H2   NC   NC
 H3   VSS   GND
 H4   W#   INBUF
 H5   VSS   GND
 H6   DQA5   Progbuf1
 H7   DQA6   Progbuf1
 J1   VDDQ   POWER
 J2   VDD   POWER
 J3   NC   NC
 J4   VDD   POWER
 J5   NC   NC
 J6   VDD   POWER
 J7   VDDQ   POWER
 K1   NC   NC
 K2   DQB5   Progbuf1
 K3   VSS   GND
 K4   CK   INBUF
 K5   VSS   GND
 K6   NC   NC
 K7   NC   NC
 L1   DQB6   Progbuf1
 L2   NC   NC
 L3   NC   NC
 L4   NC   NC
 L5   BA#   INBUF
 L6   DQA3   Progbuf1
 L7   DQA4   Progbuf1
 M1   VDDQ   POWER
 M2   DQB7   Progbuf1
 M3   VSS   GND
 M4   CKE#   INBUF
 M5   VSS   GND
 M6   NC   NC
 M7   VDDQ   POWER
 N1   DQB8   Progbuf1
 N2   NC   NC
 N3   VSS   GND
 N4   A1   INBUF
 N5   VSS   GND
 N6   DQA2   Progbuf1
 N7   NC   NC
 P1   NC   NC
 P2   DQB9   Progbuf1
 P3   VSS   GND
 P4   A0   INBUF
 P5   VSS   GND
 P6   NC   NC
 P7   DQA1   Progbuf1
 R1   NC   NC
 R2   A2   INBUF
 R3   LBO#   INBUF
 R4   VDD   POWER
 R5   FT#   INBUF
 R6   A13   INBUF
 R7   NC   NC
 T1   A21   INBUF
 T2   A10   INBUF
 T3   A11   INBUF
 T4   A20   INBUF
 T5   A12   INBUF
 T6   A19   INBUF
 T7   ZZ   INBUF
 U1   VDDQ   POWER
 U2   TMS   INBUF
 U3   TDI   INBUF
 U4   TCK   INBUF
 U5   TDO   Progbuf2
 U6   NC   NC
 U7   VDDQ   POWER
[Component]   GS8642Z36B
[Manufacturer]   GSI Technology
[Package]
|  variable   typ   min   max
R_pkg   0.2   0.1   0.5
L_pkg   3nH   1nH   5nH
C_pkg   1.5pF   1pF   3pF
[Pin]   signal_name model_name  R_pin   L_pin   C_pin
A1   VDDQ   POWER
B1   NC   NC
C1   NC   NC
D1   DQC4   Progbuf1
E1   DQC3   Progbuf1
F1   VDDQ   POWER
G1   DQC2   Progbuf1
H1   DQC1   Progbuf1
J1   VDDQ   POWER
K1   DQD1   Progbuf1
L1   DQD2   Progbuf1
M1   VDDQ   POWER
N1   DQD3   Progbuf1
P1   DQD4   Progbuf1
R1   NC   NC
T1   NC   NC
U1   VDDQ   POWER
A2   A6   INBUF
B2   E2   INBUF
C2   A5   INBUF
D2   DQC9   Progbuf1
E2   DQC8   Progbuf1
F2   DQC7   Progbuf1
G2   DQC6   Progbuf1
H2   DQC5   Progbuf1
J2   VDD   POWER
K2   DQD5   Progbuf1
L2   DQD6   Progbuf1
M2   DQD7   Progbuf1
N2   DQD8   Progbuf1
P2   DQD9   Progbuf1
R2   A2   INBUF
T2   A20   INBUF
U2   TMS   INBUF
A3   A7   INBUF
B3   A4   INBUF
C3   A3   INBUF
D3   VSS   GND
E3   VSS   GND
F3   VSS   GND
G3   BC#   INBUF
H3   VSS   GND
J3   NC   NC
K3   VSS   GND
L3   BD#   INBUF
M3   VSS   GND
N3   VSS   GND
P3   VSS   GND
R3   LBO#   INBUF
T3   A10   INBUF
U3   TDI   INBUF
A4   A18   INBUF
B4   ADV   INBUF
C4   VDD   POWER
D4   ZQ   INBUF
E4   E1#   INBUF
F4   G#   INBUF
G4   A17   INBUF
H4   W#   INBUF
J4   VDD   POWER
K4   CK   INBUF
L4   NC   NC
M4   CKE#   INBUF
N4   A1   INBUF
P4   A0   INBUF
R4   VDD   POWER
T4   A11   INBUF
U4   TCK   INBUF
A5   A8   INBUF
B5   A15   INBUF
C5   A14   INBUF
D5   VSS   GND
E5   VSS   GND
F5   VSS   GND
G5   BB#   INBUF
H5   VSS   GND
J5   NC   NC
K5   VSS   GND
L5   BA#   INBUF
M5   VSS   GND
N5   VSS   GND
P5   VSS   GND
R5   FT#   INBUF
T5   A12   INBUF
U5   TDO   Progbuf2
A6   A9   INBUF
B6   E3#   INBUF
C6   A16   INBUF
D6   DQB9   Progbuf1
E6   DQB8   Progbuf1
F6   DQB7   Progbuf1
G6   DQB6   Progbuf1
H6   DQB5   Progbuf1
J6   VDD   POWER
K6   DQA5   Progbuf1
L6   DQA6   Progbuf1
M6   DQA7   Progbuf1
N6   DQA8   Progbuf1
P6   DQA9   Progbuf1
R6   A13   INBUF
T6   A19   INBUF
U6   NC   NC
A7   VDDQ   POWER
B7   NC   NC
C7   NC   NC
D7   DQB4   Progbuf1
E7   DQB3   Progbuf1
F7   VDDQ   POWER
G7   DQB2   Progbuf1
H7   DQB1   Progbuf1
J7   VDDQ   POWER
K7   DQA1   Progbuf1
L7   DQA2   Progbuf1
M7   VDDQ   POWER
N7   DQA3   Progbuf1
P7   DQA4   Progbuf1
R7   PE#   NC
T7   ZZ   INBUF
U7   VDDQ   POWER
[Component]   GS8642Z72C
[Manufacturer]   GSI Technology
[Package]
|  variable   typ   min   max
R_pkg   0.2   0.1   0.5
L_pkg   3nH   1nH   5nH
C_pkg   1.5pF   1pF   3pF
[Pin]   signal_name model_name  R_pin   L_pin   C_pin
 A1   DQG5   Progbuf1
 A2   DQG1   Progbuf1
 A3   A13   INBUF
 A4   E2   INBUF
 A5   A14   INBUF
 A6   ADV   INBUF
 A7   A15   INBUF
 A8   E3   INBUF
 A9   A17   INBUF
 A10   DQB1   Progbuf1
 A11   DQB5   Progbuf1
 B1   DQG6   Progbuf1
 B2   DQG2   Progbuf1
 B3   BC   INBUF
 B4   BG   INBUF
 B5   NC   NC
 B6   W   INBUF
 B7   A16   INBUF
 B8   BB   INBUF
 B9   BF   INBUF
 B10   DQB2   Progbuf1
 B11   DQB6   Progbuf1
 C1   DQG7   Progbuf1
 C2   DQG3   Progbuf1
 C3   BH   INBUF
 C4   BD   INBUF
 C5   NC   NC
 C6   E1   INBUF
 C7   NC   NC
 C8   BE   INBUF
 C9   BA   INBUF
 C10   DQB3   Progbuf1
 C11   DQB7   Progbuf1
 D1   DQG8   Progbuf1
 D2   DQG4   Progbuf1
 D3   VSS   GND
 D4   NC   NC
 D5   NC   NC
 D6   G   INBUF
 D7   NC   NC
 D8   NC   NC
 D9   VSS   GND
 D10   DQB4   Progbuf1
 D11   DQB8   Progbuf1
 E1   DQG9   Progbuf1
 E2   DQC9   Progbuf1
 E3   VDDQ   POWER
 E4   VDDQ   POWER
 E5   VDD   POWER
 E6   VDD   POWER
 E7   VDD   POWER
 E8   VDDQ   POWER
 E9   VDDQ   POWER
 E10   DQF9   Progbuf1
 E11   DQB9   Progbuf1
 F1   DQC4   Progbuf1
 F2   DQC8   Progbuf1
 F3   VSS   GND
 F4   VSS   GND
 F5   VSS   GND
 F6   ZQ   INBUF
 F7   VSS   GND
 F8   VSS   GND
 F9   VSS   GND
 F10   DQF8   Progbuf1
 F11   DQF4   Progbuf1
 G1   DQC3   Progbuf1
 G2   DQC7   Progbuf1
 G3   VDDQ   POWER
 G4   VDDQ   POWER
 G5   VDD   POWER
 G6   MCH   INBUF
 G7   VDD   POWER
 G8   VDDQ   POWER
 G9   VDDQ   POWER
 G10   DQF7   Progbuf1
 G11   DQF3   Progbuf1
 H1   DQC2   Progbuf1
 H2   DQC6   Progbuf1
 H3   VSS   GND
 H4   VSS   GND
 H5   VSS   GND
 H6   MCL   INBUF
 H7   VSS   GND
 H8   VSS   GND
 H9   VSS   GND
 H10   DQF6   Progbuf1
 H11   DQF2   Progbuf1
 J1   DQC1   Progbuf1
 J2   DQC5   Progbuf1
 J3   VDDQ   POWER
 J4   VDDQ   POWER
 J5   VDD   POWER
 J6   MCH   INBUF
 J7   VDD   POWER
 J8   VDDQ   POWER
 J9   VDDQ   POWER
 J10   DQF5   Progbuf1
 J11   DQF1   Progbuf1
 K1   NC   NC
 K2   NC   NC
 K3   CK   INBUF
 K4   NC   NC
 K5   VSS   GND
 K6   MCL   INBUF
 K7   VSS   GND
 K8   NC   NC
 K9   NC   NC
 K10   NC   NC
 K11   NC   NC
 L1   DQH1   Progbuf1
 L2   DQH5   Progbuf1
 L3   VDDQ   POWER
 L4   VDDQ   POWER
 L5   VDD   POWER
 L6   FT   INBUF
 L7   VDD   POWER
 L8   VDDQ   POWER
 L9   VDDQ   POWER
 L10   DQA5   Progbuf1
 L11   DQA1   Progbuf1
 M1   DQH2   Progbuf1
 M2   DQH6   Progbuf1
 M3   VSS   GND
 M4   VSS   GND
 M5   VSS   GND
 M6   MCL   INBUF
 M7   VSS   GND
 M8   VSS   GND
 M9   VSS   GND
 M10   DQA6   Progbuf1
 M11   DQA2   Progbuf1
 N1   DQH3   Progbuf1
 N2   DQH7   Progbuf1
 N3   VDDQ   POWER
 N4   VDDQ   POWER
 N5   VDD   POWER
 N6   MCH   INBUF
 N7   VDD   POWER
 N8   VDDQ   POWER
 N9   VDDQ   POWER
 N10   DQA7   Progbuf1
 N11   DQA3   Progbuf1
 P1   DQH4   Progbuf1
 P2   DQH8   Progbuf1
 P3   VSS   GND
 P4   VSS   GND
 P5   VSS   GND
 P6   ZZ   INBUF
 P7   VSS   GND
 P8   VSS   GND
 P9   VSS   GND
 P10   DQA8   Progbuf1
 P11   DQA4   Progbuf1
 R1   DQD9   Progbuf1
 R2   DQH9   Progbuf1
 R3   VDDQ   POWER
 R4   VDDQ   POWER
 R5   VDD   POWER
 R6   VDD   POWER
 R7   VDD   POWER
 R8   VDDQ   POWER
 R9   VDDQ   POWER
 R10   DQA9   Progbuf1
 R11   DQE9   Progbuf1
 T1   DQD8   Progbuf1
 T2   DQD4   Progbuf1
 T3   VSS   GND
 T4   NC   NC
 T5   NC   NC
 T6   LBO   INBUF
 T7   NC   NC
 T8   NC   NC
 T9   VSS   GND
 T10   DQE4   Progbuf1
 T11   DQE8   Progbuf1
 U1   DQD7   Progbuf1
 U2   DQD3   Progbuf1
 U3   NC   NC
 U4   A12   INBUF
 U5   A20   INBUF
 U6   A11   INBUF
 U7   A18   INBUF
 U8   A10   INBUF
 U9   NC   NC
 U10   DQE3   Progbuf1
 U11   DQE7   Progbuf1
 V1   DQD6   Progbuf1
 V2   DQD2   Progbuf1
 V3   A9   INBUF
 V4   A8   INBUF
 V5   A7   INBUF
 V6   A1   INBUF
 V7   A6   INBUF
 V8   A5   INBUF
 V9   A4   INBUF
 V10   DQE2   Progbuf1
 V11   DQE6   Progbuf1
 W1   DQD5   Progbuf1
 W2   DQD1   Progbuf1
 W3   TMS   INBUF
 W4   TDI   INBUF
 W5   A3   INBUF
 W6   A0   INBUF
 W7   A2   INBUF
 W8   TDO   Progbuf2
 W9   TCK   INBUF
 W10   DQE1   Progbuf1
 W11   DQE5   Progbuf1
[Model Selector]   Progbuf1
VIO_2Ldriver   Low  DQ driver for VDD=3.3V VDDQ=3.3V
VIO_2Hdriver   High DQ driver for VDD=3.3V VDDQ=3.3V
VIO_3Ldriver   Low  DQ driver for VDD=3.3V VDDQ=2.5V
VIO_3Hdriver   High DQ driver for VDD=3.3V VDDQ=2.5V
VIO_4Ldriver   Low  DQ driver for VDD=2.5V VDDQ=2.5V
VIO_4Hdriver   High DQ driver for VDD=2.5V VDDQ=2.5V
VIO_5Ldriver   Low  DQ driver for VDD=2.5V VDDQ=1.8V
VIO_5Hdriver   High DQ driver for VDD=2.5V VDDQ=1.8V
VIO_6Ldriver   Low  DQ driver for VDD=1.8V VDDQ=1.8V
VIO_6Hdriver   High DQ driver for VDD=1.8V VDDQ=1.8V
[Model Selector]   IOBUF
VIO_2Hdriver   High DQ driver for VDD=3.3V VDDQ=3.3V
VIO_3Hdriver   High DQ driver for VDD=3.3V VDDQ=2.5V
VIO_4Hdriver   High DQ driver for VDD=2.5V VDDQ=2.5V
VIO_5Hdriver   High DQ driver for VDD=2.5V VDDQ=1.8V
VIO_6Hdriver   High DQ driver for VDD=1.8V VDDQ=1.8V
[Model Selector]   Progbuf2
TDO_2driver   TDO driver for VDD=3.3V VDDQ=3.3V
TDO_3driver   TDO driver for VDD=3.3V VDDQ=2.5V
TDO_4driver   TDO driver for VDD=2.5V VDDQ=2.5V
TDO_5driver   TDO driver for VDD=2.5V VDDQ=1.8V
TDO_6driver   TDO driver for VDD=1.8V VDDQ=1.8V
[Model Selector]   INBUF
INBUF3_3   INBUF driver for VDD=3.3V
INBUF2_5   INBUF driver for VDD=2.5V
INBUF1_8   INBUF driver for VDD=1.8V
| Models and submodels in the file (18): VIO_2Ldriver (I/O), VIO_2Hdriver (I/O), VIO_3Ldriver (I/O), VIO_3Hdriver (I/O), VIO_4Ldriver (I/O), VIO_4Hdriver (I/O), VIO_5Ldriver (I/O), VIO_5Hdriver (I/O), VIO_6Ldriver (I/O), VIO_6Hdriver (I/O), TDO_2driver (3-state), TDO_3driver (3-state), TDO_4driver (3-state), TDO_5driver (3-state), TDO_6driver (3-state), INBUF3_3 (Input), INBUF2_5 (Input), INBUF1_8 (Input)
